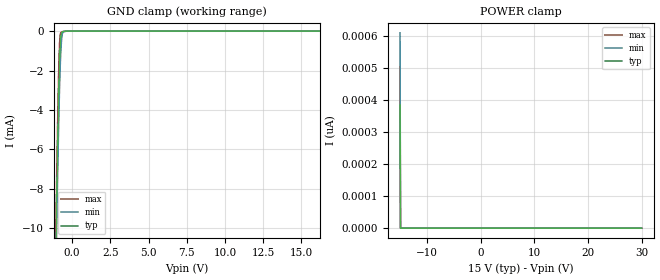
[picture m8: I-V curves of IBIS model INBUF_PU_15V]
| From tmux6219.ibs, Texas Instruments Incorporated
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| Model9
[Model]   INBUF_PU_15V
Model_type   Input
Vinl = 0.8
Vinh = 1.3
|   typ   min   max
C_comp   1.85pF   1.7pF   2.1pF
[Voltage Range]   15   13.5   16.5
[Temperature Range]   27   125   -40
[Power Clamp Reference]   15   13.5   16.5
[GND Clamp Reference]   0   0   0
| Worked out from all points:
|   GND clamp passes 1 mA (typ) near -0.80 V on its own axis
[GND Clamp]
|   Voltage   I(typ)   I(min)   I(max)
-15V      -759mA     -758.1mA   -760mA
-1.095V   -12.42mA   -13.77mA   -11.35mA
-1.05V    -10.29mA   -11.7mA    -9.178mA
-1.005V   -8.227mA   -9.688mA   -7.071mA
-915mV    -4.411mA   -5.947mA   -3.214mA
-870mV    -2.785mA   -4.298mA   -1.663mA
-825mV    -1.491mA   -2.875mA   -614.1uA
-780mV    -631.1uA   -1.743mA   -164.1uA
-735mV    -200.1uA   -926.2uA   -65.34uA
-645mV    -28.72uA   -147.5uA   -35.44uA
-375mV    -4.78uA    -1.587uA   -5.863uA
30V       0A         0A         0A
[POWER Clamp]
|   Voltage   I(typ)   I(min)   I(max)
-15V      384.9pA    610.7pA    505pA
-14.91V   0A         0A         0A
-14.87V   0A         0A         0A
30V       0A         0A         0A
